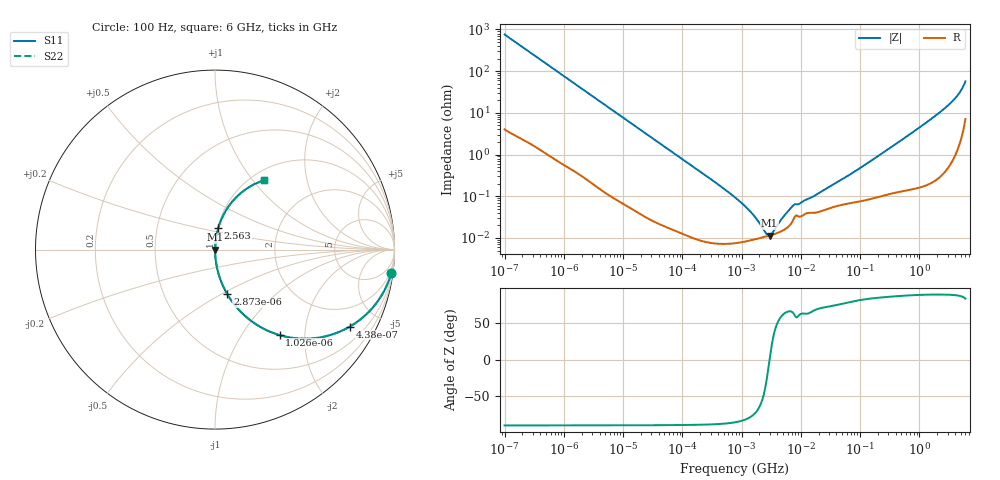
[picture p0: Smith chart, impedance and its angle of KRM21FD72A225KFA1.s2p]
!Murata Part Number: KRM21FD72A225KFA1
!These Parameters are Measured in Series Mode Connection
!Data Generated on Jan 08, 2026
!  o--ll--o
!Port1  Port2
!  o------o
!Operation Temp=25[degC], DC Bias Voltage=0[V]
!Freq. Start=100[Hz] Stop=6[GHz] 401[Steps]
# Hz S RI R 50
!Freq.(Hz) S11(Real) S11(Imag) S21(Real) S21(Imag) S12(Real) S12(Imag) S22(Real) S22(Imag)
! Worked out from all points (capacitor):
!   401 points, 100 Hz to 6 GHz, reference 50 ohm
!   read as one part in series: C = 2.09 uF near 109 Hz
!   lowest |Z| = 11.5 mohm at 2.968 MHz (marker M1)
!   S11 on the Smith chart (normalised r, x): 100 Hz: 1, -15; 438 Hz: 1.02, -3.49; 1.026 kHz: 1.01, -1.49; 2.873 kHz: 1.00, -0.54; 2.563 GHz: 1.01, +0.24; 6 GHz: 1.14, +1.14
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100  0.9823 -0.1292  0.0177 0.1292  0.0177 0.1292  0.9823 -0.1292
224  0.9191 -0.2696  0.0809 0.2696  0.0809 0.2696  0.9191 -0.2696
438  0.751 -0.429  0.249 0.429  0.249 0.429  0.751 -0.429
686  0.5545 -0.4935  0.4455 0.4935  0.4455 0.4935  0.5545 -0.4935
1026  0.3595 -0.4762  0.6405 0.4762  0.6405 0.4762  0.3595 -0.4762
2008  0.13 -0.3324  0.87 0.3324  0.87 0.3324  0.13 -0.3324
2873  0.0689 -0.2494  0.9311 0.2494  0.9311 0.2494  0.0689 -0.2494
8801  0.00841 -0.0873  0.9916 0.0873  0.9916 0.0873  0.00841 -0.0873
40335  0.000591 -0.0193  0.9994 0.0193  0.9994 0.0193  0.000591 -0.0193
774597  7.58e-05 -0.000938  0.9999 0.000938  0.9999 0.000938  7.58e-05 -0.000938
1386327  8.72e-05 -0.000432  0.9999 0.000432  0.9999 0.000432  8.72e-05 -0.000432
2594782  0.000109 -6.81e-05  0.9999 6.81e-05  0.9999 6.81e-05  0.000109 -6.81e-05
2967816  0.000115 0  0.9999 0  0.9999 0  0.000115 0
3245845  0.000119 4.51e-05  0.9999 -4.51e-05  0.9999 -4.51e-05  0.000119 4.51e-05
4856642  0.000149 0.000258  0.9999 -0.000258  0.9999 -0.000258  0.000149 0.000258
7266822  0.000254 0.000525  0.9997 -0.000525  0.9997 -0.000525  0.000254 0.000525
1.555665e7  0.000399 0.000869  0.9996 -0.000869  0.9996 -0.000869  0.000399 0.000869
7.129496e7  0.000702 0.00342  0.9993 -0.00342  0.9993 -0.00342  0.000702 0.00342
3.124326e8  0.00132 0.014  0.9987 -0.014  0.9987 -0.014  0.00132 0.014
2.562649e9  0.018 0.1193  0.982 -0.1193  0.982 -0.1193  0.018 0.1193
4.385646e9  0.0727 0.2364  0.9273 -0.2364  0.9273 -0.2364  0.0727 0.2364
6e9  0.2718 0.3868  0.7282 -0.3868  0.7282 -0.3868  0.2718 0.3868
